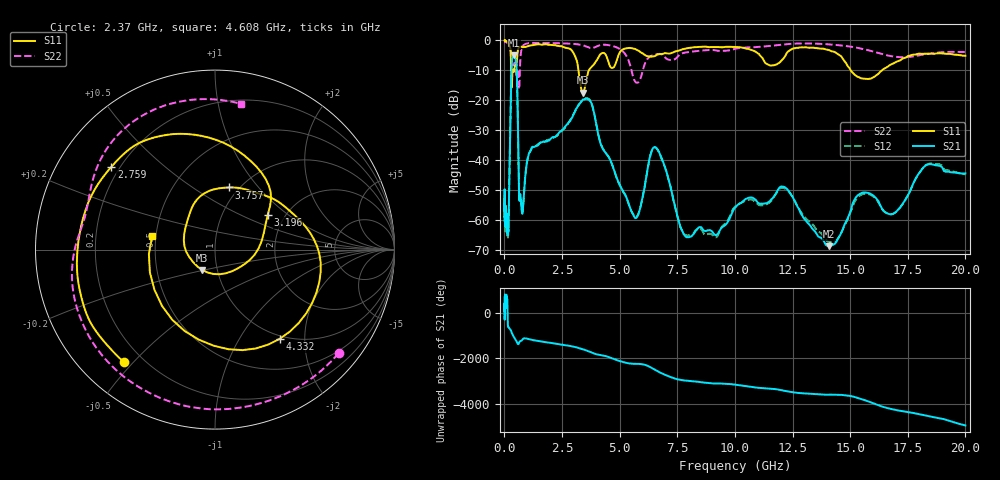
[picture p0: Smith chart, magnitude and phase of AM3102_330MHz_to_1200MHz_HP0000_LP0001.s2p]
! Date/Time: Tue, Sep 11, 2018 5:08 PM
! Network Analyzer: Agilent Technologies E8362B Rev: A.07.50.63
! Sweep from 0.010 to 20.000 GHz, 1601 Points, Sweep Type: LOG
! Power Supply: 4.950 V, 0.000 A
# Hz S DB R 50
!freq MagS11 AngS11 MagS21 AngS21 MagS12 AngS12 MagS22 AngS22
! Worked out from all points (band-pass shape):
!   1601 points, 10 MHz to 20 GHz, reference 50 ohm
!   highest |S21| = -5.00 dB at 399 MHz (marker M1); lowest = -68.7 dB at 14.07 GHz (marker M2)
!   |S21| within 3 dB of the highest: 315 MHz to 520.6 MHz (205.6 MHz wide, 49.2 % of centre)
!   lowest |S11| = -17.4 dB at 3.416 GHz (marker M3), VSWR 1.31, Z = 42.3 - j9.8 ohm
!   |S11| at or under -10 dB: 294.9 MHz to 353.9 MHz (58.92 MHz wide, 18.2 % of centre); 3.211 GHz to 3.662 GHz (450.9 MHz wide, 13.1 % of centre); 15.03 GHz to 16.38 GHz (1.351 GHz wide, 8.6 % of centre)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
!   |S22| runs from -16.3 to -0.2 dB; largest |S21 - S12| = 0.0077
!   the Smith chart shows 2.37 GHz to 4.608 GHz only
!   S11 on the Smith chart (normalised r, x): 2.37 GHz: 0.13, -0.47; 2.759 GHz: 0.17, +0.34; 3.196 GHz: 1.63, +0.72; 3.757 GHz: 0.90, +0.71; 4.332 GHz: 0.95, -1.51; 4.608 GHz: 0.48, +0.08
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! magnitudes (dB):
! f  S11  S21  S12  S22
! 10 MHz  0.0  -55.0  -54.2  -0.2
! 35.55 MHz  0.0  -60.5  -63.1  -0.4
! 126.4 MHz  -0.4  -60.7  -62.4  -0.8
! 182.2 MHz  -1.0  -60.6  -60.2  -1.2
! 304.4 MHz  -13.7  -10.0  -10.0  -6.6
! 399 MHz  -10.4  -5.0  -5.1  -8.5
! 447.2 MHz  -8.9  -5.5  -5.5  -7.4
! 765 MHz  -2.2  -57.5  -56.8  -2.4
! 1.59 GHz  -1.4  -34.0  -34.1  -0.8
! 2.37 GHz  -1.9  -30.8  -31.1  -0.9
! 2.759 GHz  -2.6  -27.7  -27.8  -1.0
! 3.196 GHz  -9.1  -21.7  -21.9  -1.3
! 3.416 GHz  -17.4  -19.7  -19.9  -1.6
! 3.757 GHz  -9.0  -20.6  -20.6  -2.5
! 4.332 GHz  -4.2  -36.9  -36.8  -1.4
! 4.608 GHz  -8.9  -40.1  -40.2  -1.7
! 5.652 GHz  -2.8  -59.1  -58.9  -13.5
! 6.58 GHz  -4.9  -35.8  -35.9  -4.6
! 7.92 GHz  -2.6  -65.7  -65.1  -3.9
! 12.09 GHz  -6.1  -48.8  -49.1  -1.4
! 14.07 GHz  -3.2  -68.7  -67.3  -1.3
! 20 GHz  -5.1  -44.4  -44.7  -3.8
